// ------------------------------------------------------------------
// File           : C:\Programmi\Siemens\NCVar Selector\pippo.awl
//
// Source File    : C:\Programmi\Siemens\NCVar Selector\pippo.var
// Generation Date: 19/11/2013  Time: 11.35.20
// ------------------------------------------------------------------

DATA_BLOCK DB  120
VERSION : 0.0


STRUCT

 C1_RP_R21_1:
   STRUCT
   SYNTAX_ID : BYTE  := B#16#82;
   bereich_u_einheit : BYTE := B#16#41;
   spalte : WORD := W#16#1;
   zeile : WORD := W#16#15;
   bausteintyp : BYTE := B#16#15;
   ZEILENANZAHL : BYTE := B#16#1;
   typ : BYTE := B#16#F;
   laenge : BYTE := B#16#8;
   END_STRUCT ;

 C1_RP_R31_1:
   STRUCT
   SYNTAX_ID : BYTE  := B#16#82;
   bereich_u_einheit : BYTE := B#16#41;
   spalte : WORD := W#16#1;
   zeile : WORD := W#16#1F;
   bausteintyp : BYTE := B#16#15;
   ZEILENANZAHL : BYTE := B#16#1;
   typ : BYTE := B#16#F;
   laenge : BYTE := B#16#8;
   END_STRUCT ;

 C1_RP_R32_1:
   STRUCT
   SYNTAX_ID : BYTE  := B#16#82;
   bereich_u_einheit : BYTE := B#16#41;
   spalte : WORD := W#16#1;
   zeile : WORD := W#16#20;
   bausteintyp : BYTE := B#16#15;
   ZEILENANZAHL : BYTE := B#16#1;
   typ : BYTE := B#16#F;
   laenge : BYTE := B#16#8;
   END_STRUCT ;

 C1_RP_R41_1:
   STRUCT
   SYNTAX_ID : BYTE  := B#16#82;
   bereich_u_einheit : BYTE := B#16#41;
   spalte : WORD := W#16#1;
   zeile : WORD := W#16#29;
   bausteintyp : BYTE := B#16#15;
   ZEILENANZAHL : BYTE := B#16#1;
   typ : BYTE := B#16#F;
   laenge : BYTE := B#16#8;
   END_STRUCT ;

 C1_RP_R12_1:
   STRUCT
   SYNTAX_ID : BYTE  := B#16#82;
   bereich_u_einheit : BYTE := B#16#41;
   spalte : WORD := W#16#1;
   zeile : WORD := W#16#C;
   bausteintyp : BYTE := B#16#15;
   ZEILENANZAHL : BYTE := B#16#1;
   typ : BYTE := B#16#F;
   laenge : BYTE := B#16#8;
   END_STRUCT ;

 C1_RP_R13_1:
   STRUCT
   SYNTAX_ID : BYTE  := B#16#82;
   bereich_u_einheit : BYTE := B#16#41;
   spalte : WORD := W#16#1;
   zeile : WORD := W#16#D;
   bausteintyp : BYTE := B#16#15;
   ZEILENANZAHL : BYTE := B#16#1;
   typ : BYTE := B#16#F;
   laenge : BYTE := B#16#8;
   END_STRUCT ;

 C1_RP_R14_1:
   STRUCT
   SYNTAX_ID : BYTE  := B#16#82;
   bereich_u_einheit : BYTE := B#16#41;
   spalte : WORD := W#16#1;
   zeile : WORD := W#16#E;
   bausteintyp : BYTE := B#16#15;
   ZEILENANZAHL : BYTE := B#16#1;
   typ : BYTE := B#16#F;
   laenge : BYTE := B#16#8;
   END_STRUCT ;

 C1_RP_R15_1:
   STRUCT
   SYNTAX_ID : BYTE  := B#16#82;
   bereich_u_einheit : BYTE := B#16#41;
   spalte : WORD := W#16#1;
   zeile : WORD := W#16#F;
   bausteintyp : BYTE := B#16#15;
   ZEILENANZAHL : BYTE := B#16#1;
   typ : BYTE := B#16#F;
   laenge : BYTE := B#16#8;
   END_STRUCT ;

 C2_RP_R21_1:
   STRUCT
   SYNTAX_ID : BYTE  := B#16#82;
   bereich_u_einheit : BYTE := B#16#42;
   spalte : WORD := W#16#1;
   zeile : WORD := W#16#15;
   bausteintyp : BYTE := B#16#15;
   ZEILENANZAHL : BYTE := B#16#1;
   typ : BYTE := B#16#F;
   laenge : BYTE := B#16#8;
   END_STRUCT ;

 C2_RP_R31_1:
   STRUCT
   SYNTAX_ID : BYTE  := B#16#82;
   bereich_u_einheit : BYTE := B#16#42;
   spalte : WORD := W#16#1;
   zeile : WORD := W#16#1F;
   bausteintyp : BYTE := B#16#15;
   ZEILENANZAHL : BYTE := B#16#1;
   typ : BYTE := B#16#F;
   laenge : BYTE := B#16#8;
   END_STRUCT ;

 C2_RP_R32_1:
   STRUCT
   SYNTAX_ID : BYTE  := B#16#82;
   bereich_u_einheit : BYTE := B#16#42;
   spalte : WORD := W#16#1;
   zeile : WORD := W#16#20;
   bausteintyp : BYTE := B#16#15;
   ZEILENANZAHL : BYTE := B#16#1;
   typ : BYTE := B#16#F;
   laenge : BYTE := B#16#8;
   END_STRUCT ;

 C2_RP_R41_1:
   STRUCT
   SYNTAX_ID : BYTE  := B#16#82;
   bereich_u_einheit : BYTE := B#16#42;
   spalte : WORD := W#16#1;
   zeile : WORD := W#16#29;
   bausteintyp : BYTE := B#16#15;
   ZEILENANZAHL : BYTE := B#16#1;
   typ : BYTE := B#16#F;
   laenge : BYTE := B#16#8;
   END_STRUCT ;

 C2_RP_R12_1:
   STRUCT
   SYNTAX_ID : BYTE  := B#16#82;
   bereich_u_einheit : BYTE := B#16#42;
   spalte : WORD := W#16#1;
   zeile : WORD := W#16#C;
   bausteintyp : BYTE := B#16#15;
   ZEILENANZAHL : BYTE := B#16#1;
   typ : BYTE := B#16#F;
   laenge : BYTE := B#16#8;
   END_STRUCT ;

 C2_RP_R13_1:
   STRUCT
   SYNTAX_ID : BYTE  := B#16#82;
   bereich_u_einheit : BYTE := B#16#42;
   spalte : WORD := W#16#1;
   zeile : WORD := W#16#D;
   bausteintyp : BYTE := B#16#15;
   ZEILENANZAHL : BYTE := B#16#1;
   typ : BYTE := B#16#F;
   laenge : BYTE := B#16#8;
   END_STRUCT ;

 C2_RP_R14_1:
   STRUCT
   SYNTAX_ID : BYTE  := B#16#82;
   bereich_u_einheit : BYTE := B#16#42;
   spalte : WORD := W#16#1;
   zeile : WORD := W#16#E;
   bausteintyp : BYTE := B#16#15;
   ZEILENANZAHL : BYTE := B#16#1;
   typ : BYTE := B#16#F;
   laenge : BYTE := B#16#8;
   END_STRUCT ;

 C2_RP_R15_1:
   STRUCT
   SYNTAX_ID : BYTE  := B#16#82;
   bereich_u_einheit : BYTE := B#16#42;
   spalte : WORD := W#16#1;
   zeile : WORD := W#16#F;
   bausteintyp : BYTE := B#16#15;
   ZEILENANZAHL : BYTE := B#16#1;
   typ : BYTE := B#16#F;
   laenge : BYTE := B#16#8;
   END_STRUCT ;

 END_STRUCT ;

BEGIN
END_DATA_BLOCK
